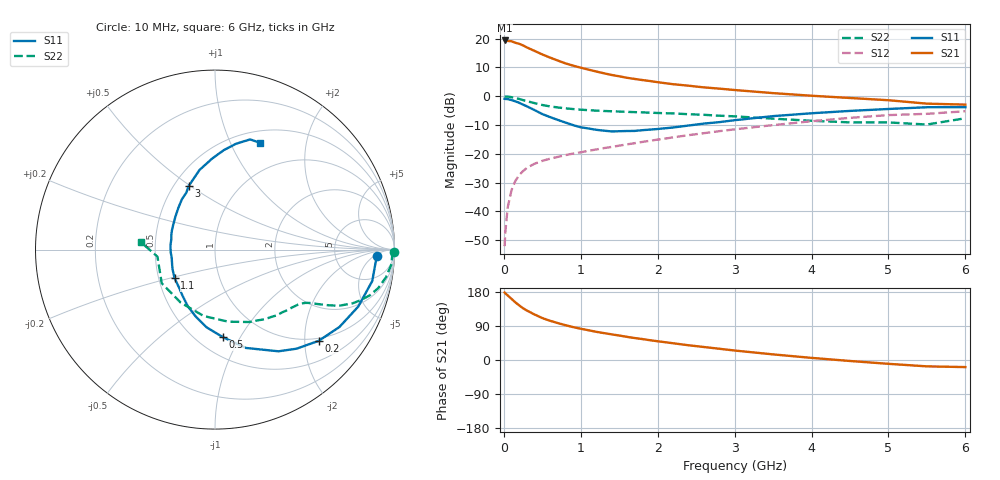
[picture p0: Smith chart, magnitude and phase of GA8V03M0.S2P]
! Infineon Technologies  Discrete & RF Semiconductors
! BF775
! Si NPN RF Bipolar Junction Transistor in SOT23
! VCE = 8 V  IC = 3 mA
! Common Emitter S-Parameters:  May  1996
# GHz  S  MA  R  50
!  f  S11  S21  S12  S22
! GHz  MAG  ANG  MAG  ANG  MAG  ANG  MAG  ANG
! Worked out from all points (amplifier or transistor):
!   36 points, 10 MHz to 6 GHz, reference 50 ohm
!   highest |S21| = 19.4 dB at 10 MHz (marker M1)
!   |S21| within 3 dB of that: start of sweep to 347.2 MHz
!   unconditionally stable (mu >= 1): 1.051 GHz to 3.127 GHz
!   at 250 MHz: K = 0.35, MSG = 21.8 dB, |S12| = -26.0 dB
!   at 1.4 GHz: K = 1.10, MAG = 10.5 dB, |S12| = -17.6 dB
!   at 6 GHz: K = 0.92, MSG = 1.2 dB, |S12| = -5.2 dB
!   S11 on the Smith chart (normalised r, x): 10 MHz: 17, -7; 200 MHz: 0.93, -2.33; 500 MHz: 0.66, -0.85; 1.1 GHz: 0.61, -0.21; 3 GHz: 0.59, +0.49; 6 GHz: 0.64, +1.30
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0.01  0.902 -2.3  9.298 178.0  0.0025 88.0  0.9977 -0.8
0.02  0.8978 -4.5  9.094 175.8  0.0045 87.0  0.9879 -1.9
0.05  0.8935 -11.3  9.132 170.4  0.0117 83.5  0.9867 -4.7
0.1  0.8589 -21.7  8.994 161.3  0.0235 78.2  0.9652 -9.2
0.15  0.8164 -31.9  8.47 152.0  0.0339 72.5  0.9342 -13.3
0.2  0.7698 -41.3  8.131 144.0  0.043 68.0  0.8987 -16.5
0.25  0.7154 -50.5  7.624 136.6  0.0503 64.3  0.8569 -19.3
0.3  0.6681 -58.0  7.024 130.4  0.0573 61.3  0.8217 -21.4
0.4  0.5742 -72.6  6.122 120.1  0.0675 56.7  0.7598 -24.3
0.5  0.4907 -84.7  5.313 110.6  0.0756 54.5  0.7053 -26.1
0.6  0.4354 -96.2  4.69 103.6  0.0824 53.1  0.6666 -27.3
0.7  0.3888 -105.9  4.172 97.5  0.0886 52.5  0.6397 -28.2
0.8  0.3504 -115.6  3.727 91.9  0.095 52.1  0.6173 -28.9
0.9  0.3154 -124.8  3.398 86.8  0.1012 52.4  0.5995 -29.7
1.1  0.276 -144.5  2.899 78.5  0.113 53.2  0.573 -31.5
1.6  0.2493 174.9  2.091 61.1  0.1462 54.4  0.5359 -37.1
2.2  0.2868 140.4  1.619 44.2  0.1931 54.1  0.5033 -46.6
3  0.3839 112.4  1.283 25.0  0.2664 50.0  0.4479 -64.3
3.5  0.452 101.0  1.133 14.8  0.3156 45.5  0.4084 -79.6
4.5  0.5567 84.9  0.933 -2.6  0.4221 33.8  0.3519 -122.9
5.5  0.6445 72.3  0.744 -16.8  0.4955 18.0  0.3231 -173.0
6  0.6456 67.0  0.716 -18.7  0.5491 13.6  0.4153 174.2
